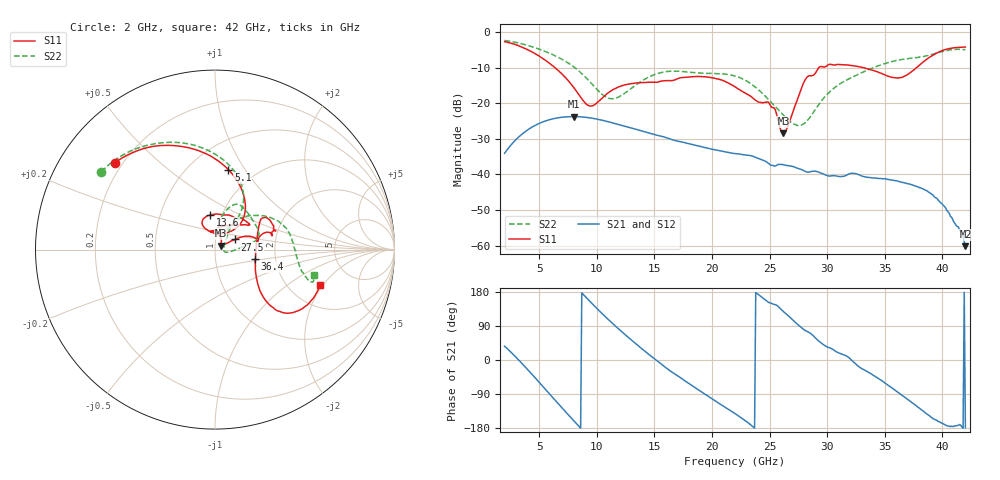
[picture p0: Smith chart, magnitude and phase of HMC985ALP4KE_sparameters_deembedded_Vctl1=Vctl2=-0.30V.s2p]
!s2p File: Measurements: S11, S21, S12, S22
# GHz S dB R 50.0
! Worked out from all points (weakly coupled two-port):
!   401 points, 2 GHz to 42 GHz, reference 50 ohm
!   highest |S21| = -23.71 dB at 8 GHz (marker M1); lowest = -60.2 dB at 42 GHz (marker M2)
!   lowest |S11| = -28.4 dB at 26.2 GHz (marker M3), VSWR 1.08, Z = 53.1 + j2.4 ohm
!   |S11| at or under -10 dB: 6.39 GHz to 29.27 GHz (22.88 GHz wide, 128 % of centre); 33.2 GHz to 37.74 GHz (4.539 GHz wide, 12.8 % of centre)
!   |S22| runs from -26.2 to -2.3 dB; largest |S21 - S12| = 0.00014
!   S11 on the Smith chart (normalised r, x): 2 GHz: 0.17, +0.36; 5.1 GHz: 0.76, +0.84; 13.6 GHz: 0.88, +0.35; 27.5 GHz: 1.24, +0.14; 36.4 GHz: 1.57, -0.17; 42 GHz: 2.93, -1.90
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2  -2.62 139.1  -34.05 36.4  -34.05 36.4  -2.30 145.5
3.5  -4.17 110.8  -28.69 -8.9  -28.70 -8.9  -3.26 121.7
5.1  -6.91 80.5  -25.50 -62.2  -25.51 -62.2  -4.85 97.3
8  -15.52 45.5  -23.71 -160.2  -23.72 -160.2  -9.73 60.7
8.7  -18.73 54.7  -23.81 177.0  -23.82 177.0  -11.64 56.0
9.6  -20.70 88.8  -24.18 148.6  -24.18 148.6  -14.60 54.3
11.2  -16.56 116.9  -25.35 101.1  -25.35 101.1  -18.67 70.3
13.6  -14.21 98.4  -27.47 37.5  -27.47 37.5  -14.37 78.0
15.4  -13.92 73.5  -29.08 -5.8  -29.08 -5.8  -11.49 68.3
19.4  -12.51 35.7  -32.44 -90.3  -32.44 -90.3  -11.53 34.6
22  -15.33 53.1  -34.13 -141.4  -34.13 -141.3  -12.31 14.1
25  -20.09 94.8  -37.18 150.9  -37.19 150.9  -19.23 -1.6
26.2  -28.37 36.3  -37.28 127.9  -37.29 127.9  -23.29 -12.7
27.5  -18.16 27.1  -38.35 92.2  -38.32 92.2  -26.19 -1.0
28.1  -13.31 19.6  -39.16 77.9  -39.12 77.7  -25.44 19.5
28.7  -12.19 11.9  -39.11 66.7  -39.14 66.7  -23.02 36.4
31.1  -9.12 23.2  -40.63 17.5  -40.60 17.8  -14.53 54.9
33.3  -10.08 33.7  -40.70 -27.5  -40.71 -27.4  -10.96 42.0
35.4  -12.45 12.0  -41.46 -68.9  -41.49 -69.0  -8.45 25.7
36.4  -12.76 -13.2  -42.15 -90.7  -42.12 -90.8  -7.68 17.1
39.6  -5.71 -42.8  -47.04 -161.6  -47.13 -160.7  -5.77 -15.7
42  -4.15 -18.8  -60.18 -179.0  -60.07 179.4  -4.91 -14.6
